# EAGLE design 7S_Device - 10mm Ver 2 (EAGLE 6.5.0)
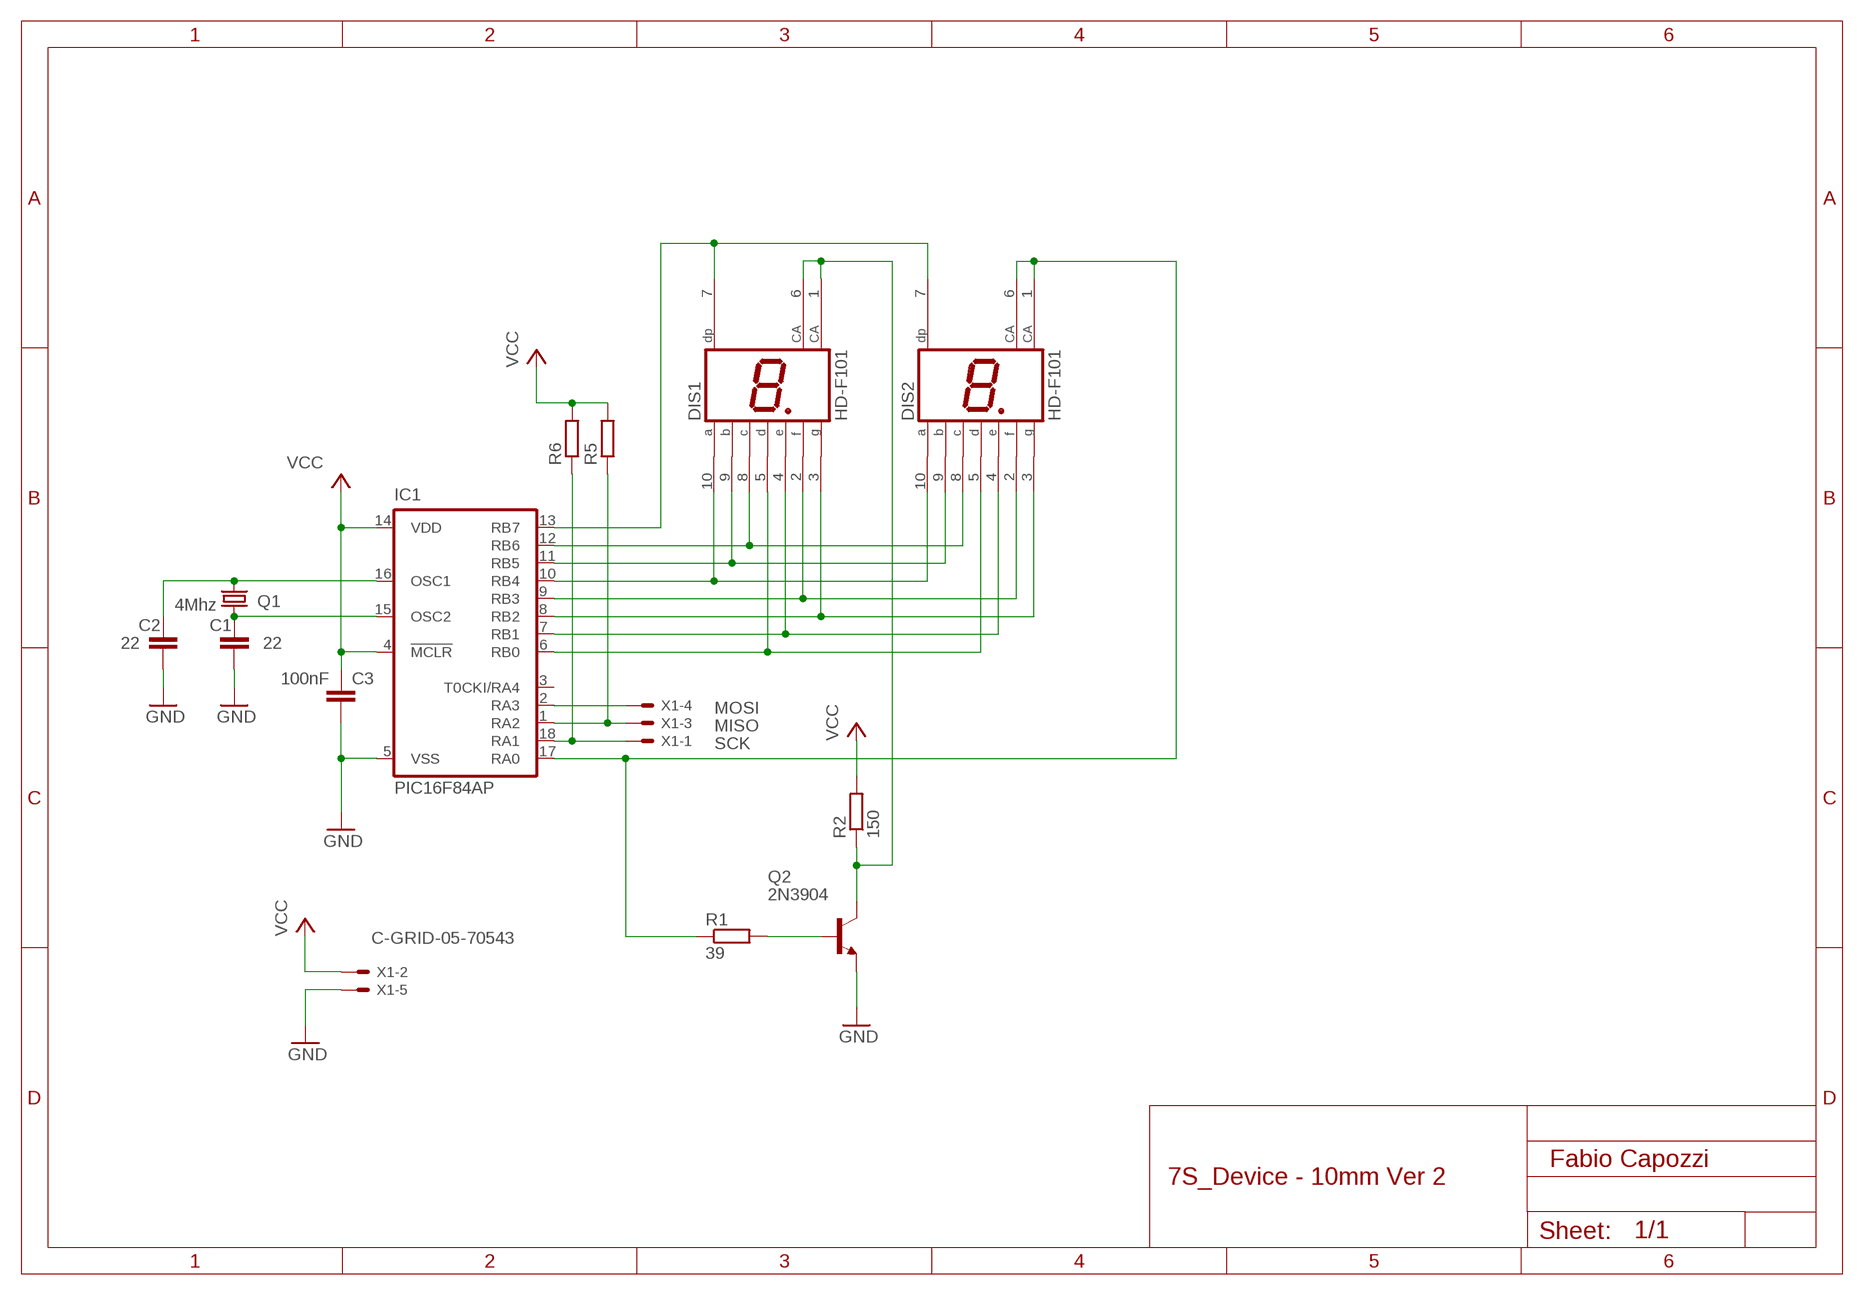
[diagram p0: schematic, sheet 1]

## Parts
C1  22  C5/2.5  [C5B2.5]
C2  22  C5/2.5  [C5B2.5]
C3  100nF  C5/2.5  [C5B2.5]
DIS1  HD-F101  [HDSP-E]
DIS2  HD-F101  [HDSP-E]
IC1  PIC16F84AP  [DIL18]
Q1  4Mhz  CRYSTALHC49U-V  [HC49U-V]
Q2  2N3904  BC489  [TO92-EBC]
R1  39  R-EU_0204/7  [0204/7]
R2  150  R-EU_0204/7  [0204/7]
R5  R-EU_0204/7  [0204/7]
R6  R-EU_0204/7  [0204/7]
X1  C-GRID-05-70543  [70543-05]

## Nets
GND: C1.2 C2.2 C3.2 IC1.5(VSS) Q2.E X1.5
N$1: C2.1 IC1.16(OSC1) Q1.2
N$2: C1.1 IC1.15(OSC2) Q1.1
N$3: DIS1.5(D) DIS2.5(D) IC1.6(RB0)
N$4: DIS1.4(E) DIS2.4(E) IC1.7(RB1)
N$5: DIS1.3(G) DIS2.3(G) IC1.8(RB2)
N$6: DIS1.2(F) DIS2.2(F) IC1.9(RB3)
N$7: DIS1.10(A) DIS2.10(A) IC1.10(RB4)
N$8: DIS1.9(B) DIS2.9(B) IC1.11(RB5)
N$9: DIS1.8(C) DIS2.8(C) IC1.12(RB6)
N$10: DIS1.7(DP) DIS2.7(DP) IC1.13(RB7)
N$11: DIS2.1(CA) DIS2.6(CA) IC1.17(RA0) R1.1
N$12: Q2.B R1.2
N$13: DIS1.1(CA) DIS1.6(CA) Q2.C R2.1
N$15: IC1.18(RA1) R6.1 X1.1
N$18: IC1.1(RA2) R5.1 X1.3
N$19: IC1.2(RA3) X1.4
VCC: C3.1 IC1.4(!MCLR) IC1.14(VDD) R2.2 R5.2 R6.2 X1.2
Unconnected: IC1.3(T0CKI/RA4)

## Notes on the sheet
- MOSI
- MISO
- SCK
- Fabio Capozzi

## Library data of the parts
C1-C3 = capacitor-wima:C: CAPACITOR
DIS1 DIS2 = display-hp:HD-F101: LED DISPLAY 1-character 7 segment, decimal point right; OC_FARNELL: unknown; OC_NEWARK: unknown
IC1 = microchip:PIC16F8*: MICROCONTROLLER 8-Bit PIC16F8X Family - CMOS Flash/EEPROM Pin Compatible : PIC16F83, PIC16CR83, PIC16F84A, PIC16CR84 see also PIC16C*; MF: MICROCHIP; MPN: PIC16F84A-04I/P; OC_FARNELL: 9760865; OC_NEWARK: 69K7635
Q1 = crystal:CRYSTAL: CRYSTAL; OC_FARNELL: 1666969; OC_NEWARK: unknown
Q2 = transistor-npn:BC489*: NPN Transistor
R1 R2 R5 R6 = rcl:R-EU_: RESISTOR, European symbol
X1 = con-molex:C-GRID-05: CONNECTOR wire to board 2.54 mm (0.100") pitch header; OC_FARNELL: unknown; OC_NEWARK: unknown

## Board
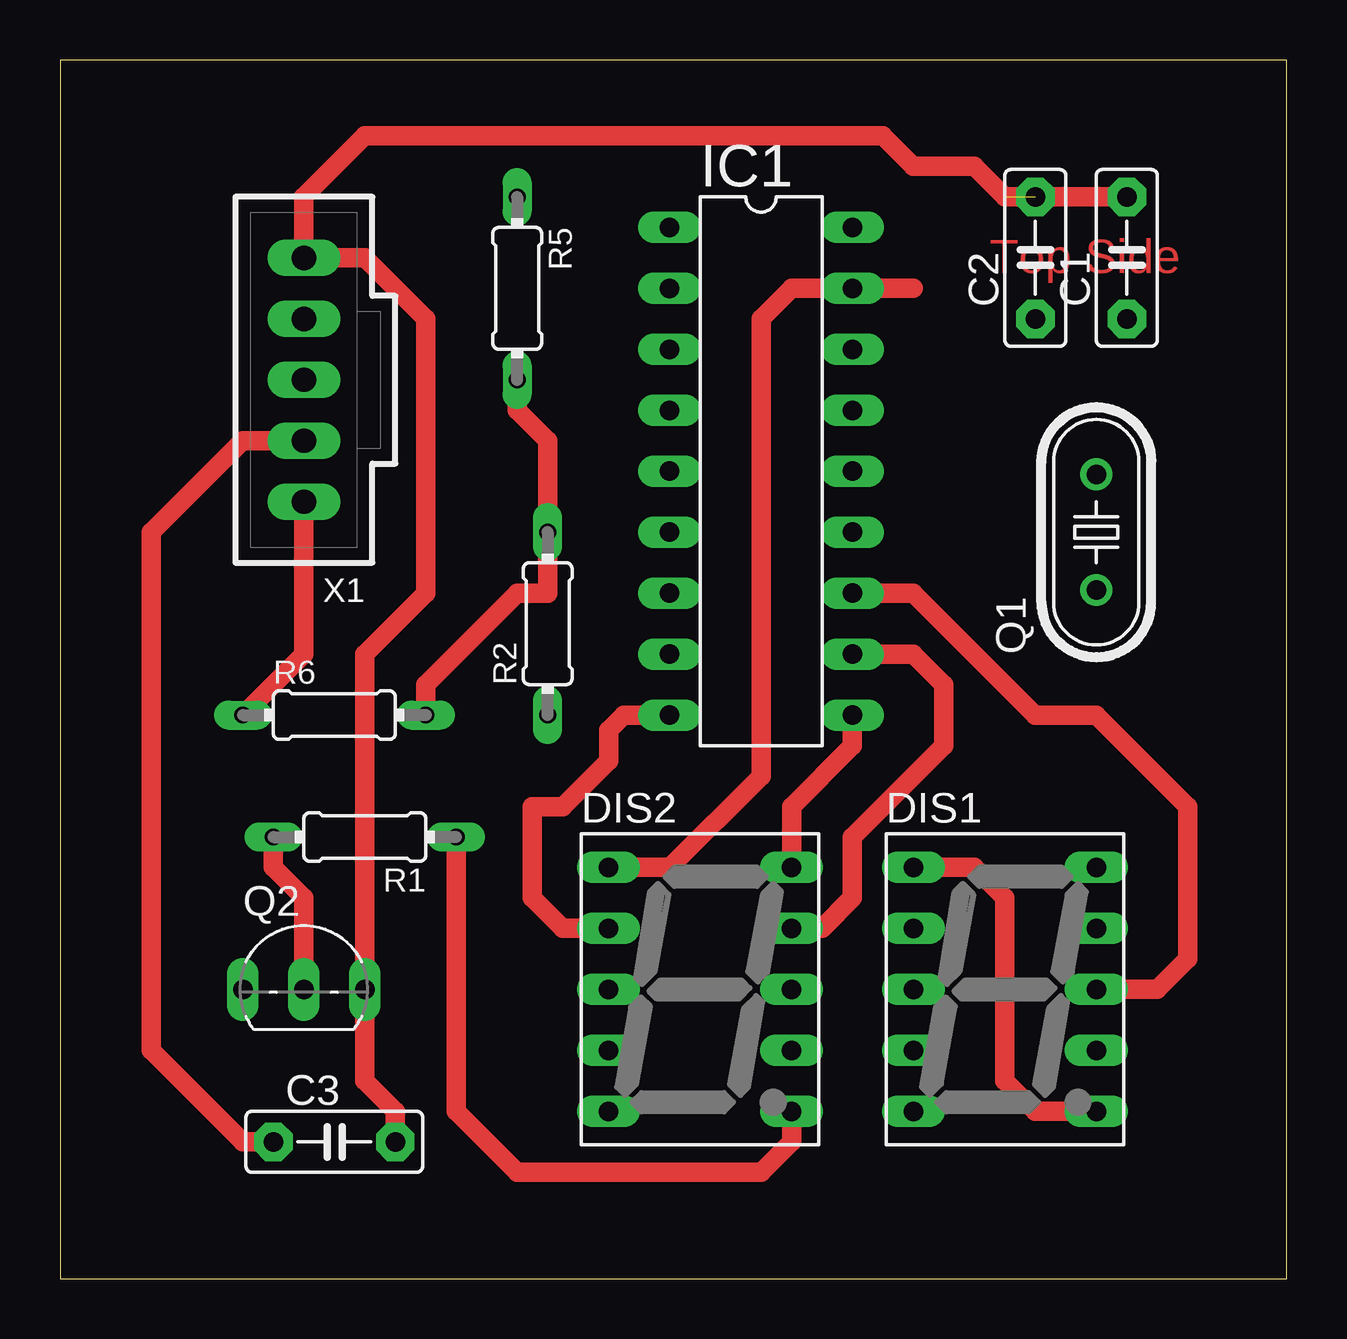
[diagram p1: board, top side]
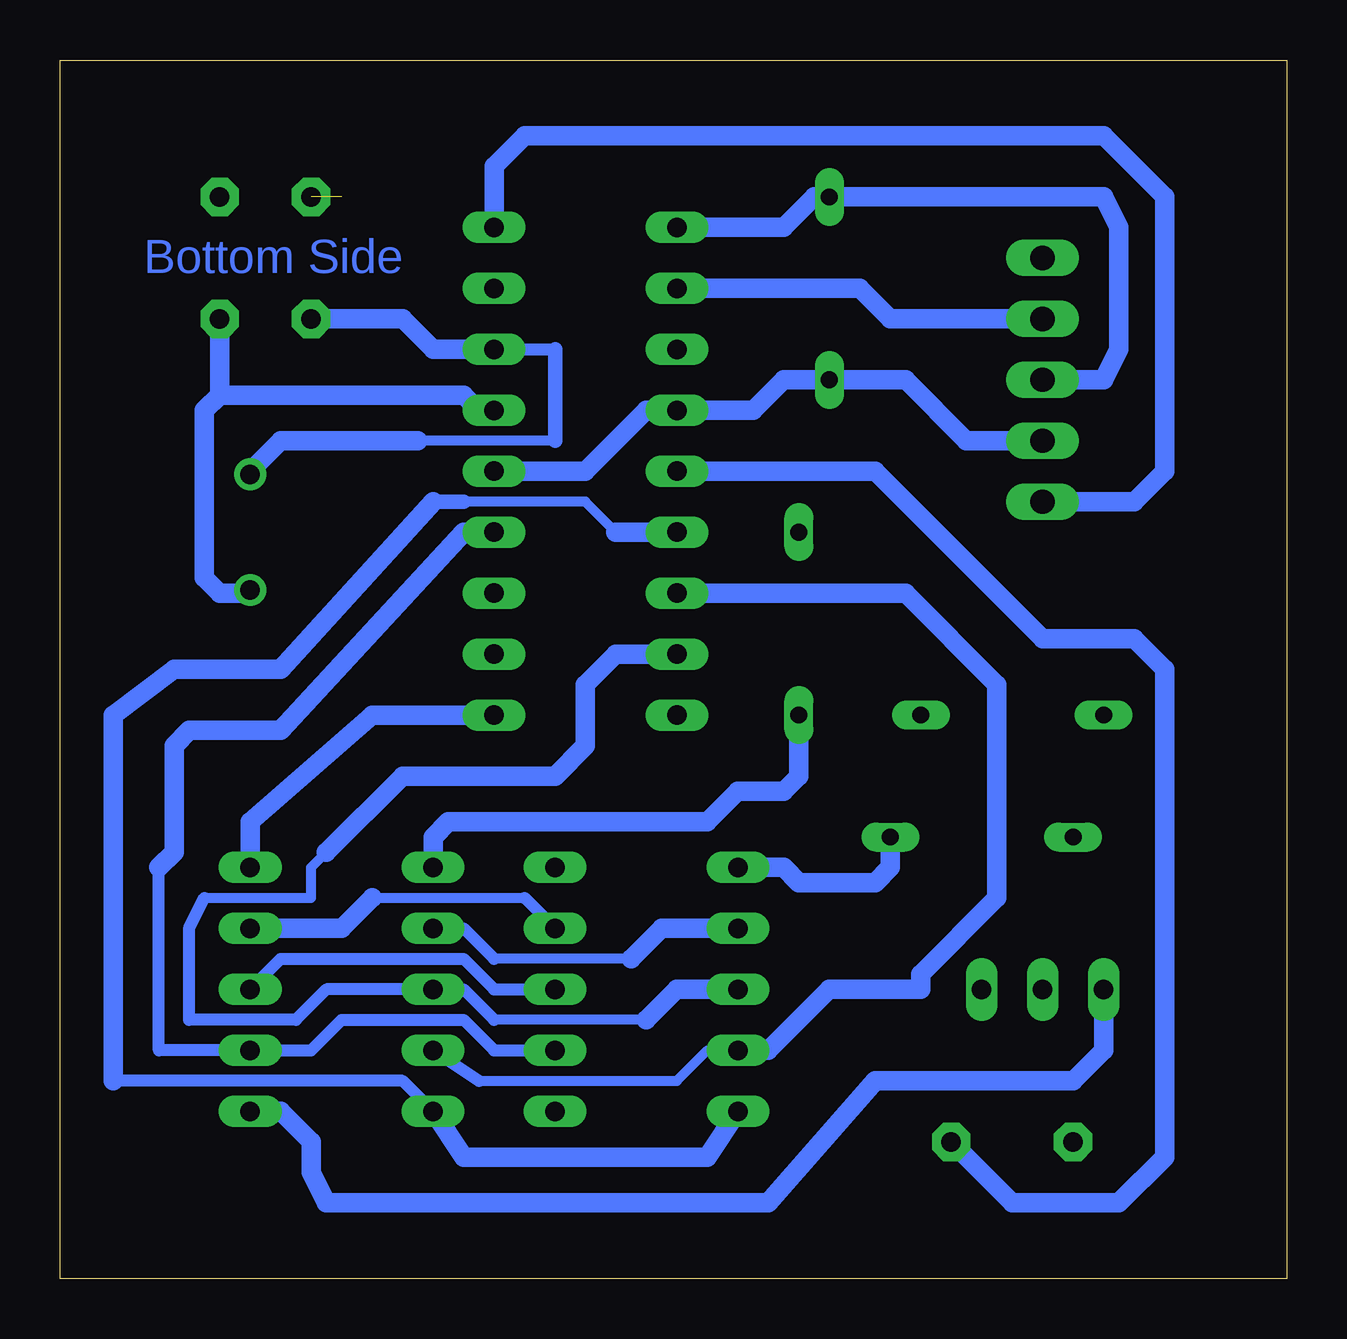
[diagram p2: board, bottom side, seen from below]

Size 51.11 x 50.79 mm. Coordinates in mm from the lower left corner, seen from the top.
Outline: 0,0 51.11,0 51.11,50.79 0,50.79 0,0
Copper layers (1*16): Top 0.035mm / dielectric 1.5mm / Bottom 0.035mm
Design rules "default *": minimum track width 20mil, minimum drill 24mil, track to track 8mil, track to pad 8mil, pad to pad 8mil, via to via 8mil, smd to smd 8mil, copper to edge 40mil, drill to drill 8mil, minimum pad ring 10mil, minimum via ring 8mil, stop-mask expansion 4mil, vias tented up to drill 0mil, thermal gap 10mil
tRestrict: area 40.6,26 to 45.7,36.2; area 26.7,22.2 to 31.8,45.1; area 36.8,5.7 to 41.9,18.4; area 24.1,5.7 to 29.2,18.4

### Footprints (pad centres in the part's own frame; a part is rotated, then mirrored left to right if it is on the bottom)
C5B2.5 = drill 0.813 pad 1.6 octagon: 1 -2.54,0; 2 2.54,0
HDSP-E = drill 0.813 long: 1 -3.81,5.08; 2 -3.81,2.54; 3 -3.81,0; 4 -3.81,-2.54; 5 -3.81,-5.08; 6 3.81,-5.08; 7 3.81,-2.54; 8 3.81,0; 9 3.81,2.54; 10 3.81,5.08
DIL18 = drill 0.813 long: 1 -10.16,-3.81; 2 -7.62,-3.81; 3 -5.08,-3.81; 4 -2.54,-3.81; 5 0,-3.81; 6 2.54,-3.81; 7 5.08,-3.81; 8 7.62,-3.81; 9 10.16,-3.81; 10 10.16,3.81; 11 7.62,3.81; 12 5.08,3.81; 13 2.54,3.81; 14 0,3.81; 15 -2.54,3.81; 16 -5.08,3.81; 17 -7.62,3.81; 18 -10.16,3.81
HC49U-V = drill 0.813: 1 -2.413,0; 2 2.413,0
TO92-EBC = drill 0.813 long: B 0,-1.27; C -2.54,-1.27; E 2.54,-1.27
0204/7 = drill 0.7 pad 1.016 long: 1 -3.81,0; 2 3.81,0
70543-05 = drill 1.016 long: 1 -5.08,0; 2 -2.54,0; 3 0,0; 4 2.54,0; 5 5.08,0

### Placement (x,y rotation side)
C1  44.45,42.54 90 top
C2  40.64,42.54 90 top
C3  11.43,5.71 0 top
DIS1  39.37,12.06 0 top
DIS2  26.67,12.06 0 top
IC1  29.21,33.66 270 top
Q1  43.18,31.12 90 top
Q2  10.16,13.33 0 top
R1  12.7,18.42 180 top
R2  20.32,27.31 90 top
R5  19.05,41.27 270 top
R6  11.43,23.5 0 top
X1  10.16,37.46 90 top

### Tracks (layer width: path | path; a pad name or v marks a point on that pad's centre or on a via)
GND  (1 unrouted)
  Top 0.813: C3.2 13.97,6.98 12.7,8.26 Q2.E 12.7,26.04 15.24,28.58 15.24,40 12.7,42.54 X1.5 10.16,45.09 12.7,47.62 34.29,47.62 35.56,46.35 38.1,46.35 39.37,45.09 C1.2
  Bottom 0.813: C3.2 11.43,3.17 6.98,3.17 5.08,5.08 5.08,25.4 6.35,26.67 10.16,26.67 17.14,33.66 IC1.5
N$1
  Bottom 0.406: 30.48,34.92 36.2,34.92
  Bottom 0.508: IC1.16 30.48,38.73 | 43.18,33.66 Q1.2
  Bottom 0.61: 30.48,38.73 30.48,34.92
  Bottom 0.813: 43.18,33.66 41.91,34.92 36.2,34.92 | IC1.16 35.56,38.73 36.83,40 C2.1
N$2
  Bottom 0.813: IC1.15 33.66,36.2 34.29,36.83 44.45,36.83 | C1.1 44.45,36.83 | 44.45,36.83 45.09,36.2 45.09,29.21 44.45,28.58 43.31,28.58 Q1.1
N$3
  Bottom 0.406: 27.94,31.12 29.21,32.38 34.29,32.38
  Bottom 0.508: 48.9,8.26 36.83,8.26 DIS1.5
  Bottom 0.61: 34.29,32.38 35.56,32.38
  Bottom 0.813: DIS2.5 24.13,5.08 34.29,5.08 DIS1.5 | 35.56,32.38 41.91,25.4 46.36,25.4 48.9,23.5 48.9,8.26 | IC1.6 27.94,31.12
N$4
  Bottom 0.406: 33.66,8.26 25.4,8.26 24.13,9.53 DIS2.4
  Bottom 0.508: DIS1.4 33.66,8.26
  Bottom 0.813: DIS2.4 21.59,9.53 19.05,12.06 15.24,12.06 15.24,12.7 12.06,15.88 12.06,24.77 15.88,28.58 IC1.7
N$5
  Bottom 0.406: 45.09,15.88 40.64,15.88 40.64,17.15 40.01,17.78 | 26.67,10.79 33.02,10.79
  Bottom 0.508: 33.02,10.79 34.29,12.06 DIS1.3 40.01,12.06 41.27,10.79 45.72,10.79 45.72,14.61 45.09,15.88
  Bottom 0.813: 40.01,17.78 36.83,20.96 30.48,20.96 29.21,22.23 29.21,24.77 27.94,26.04 IC1.8 | DIS2.3 25.4,12.06 26.67,10.79
N$6
  Top 0.813: DIS2.2 20.95,14.61 19.69,15.88 19.69,19.69 20.95,19.69 22.86,21.59 22.86,22.86 23.49,23.5 IC1.9
  Bottom 0.406: 27.3,13.33 33.02,13.33
  Bottom 0.508: 33.02,13.33 34.29,14.61 DIS1.2
  Bottom 0.813: DIS2.2 26.03,14.61 27.3,13.33
N$7
  Top 0.813: DIS2.10 30.48,19.69 33.02,22.23 IC1.10
  Bottom 0.813: IC1.10 38.1,23.5 43.18,19.05 DIS1.10
N$8
  Top 0.813: DIS2.9 31.75,14.61 33.02,15.88 33.02,18.42 36.83,22.23 36.83,24.77 35.56,26.04 IC1.11
  Bottom 0.406: 38.1,15.88 31.75,15.88
  Bottom 0.508: 31.75,15.88 DIS2.9 | DIS1.9 41.91,14.61
  Bottom 0.813: 41.91,14.61 39.37,14.61 38.1,15.88
N$9
  Top 0.813: IC1.12 35.56,28.58 40.64,23.5 43.18,23.5 46.99,19.69 46.99,13.33 45.72,12.06 DIS1.8
  Bottom 0.508: DIS2.8 33.02,12.06 34.29,13.33 41.91,13.33 DIS1.8
N$10
  Bottom 0.508: DIS2.7 33.02,9.53 34.29,10.79 39.37,10.79 40.64,9.53 DIS1.7 46.99,9.53 46.99,17.15
  Bottom 0.813: IC1.13 34.29,31.12 41.91,22.86 45.72,22.86 46.36,22.23 46.36,17.78 46.99,17.15
N$11
  Top 0.813: DIS2.1 25.4,17.15 29.21,20.96 29.21,40 30.48,41.27 IC1.17 35.56,41.27 | R1.1 16.51,6.98 19.05,4.45 29.21,4.45 30.48,5.71 DIS2.6
  Bottom 0.813: DIS2.1 20.95,17.15 20.32,16.51 17.14,16.51 16.51,17.15 R1.1
N$12
  Top 0.813: R1.2 8.89,17.15 10.16,15.88 Q2.B
N$13
  Top 0.813: DIS1.1 38.1,17.15 39.37,15.88 39.37,8.26 40.64,6.98 DIS1.6
  Bottom 0.813: Q2.C 7.62,9.53 8.89,8.26 17.14,8.26 21.59,3.17 40.01,3.17 40.64,4.45 40.64,5.71 41.91,6.98 DIS1.6 | R2.1 20.32,20.96 20.95,20.32 22.86,20.32 24.13,19.05 34.92,19.05 35.56,18.42 DIS1.1
N$15
  Top 0.813: X1.1 10.16,26.04 R6.1
  Bottom 0.813: IC1.18 33.02,46.35 31.75,47.62 7.62,47.62 5.08,45.09 5.08,33.66 6.35,32.38 X1.1
N$18
  Bottom 0.813: X1.3 7.62,37.46 6.98,38.73 6.98,43.81 7.62,45.09 R5.1 19.69,45.09 20.95,43.81 IC1.1
N$19
  Bottom 0.813: X1.4 16.51,40 17.78,41.27 IC1.2
VCC
  Top 0.813: X1.2 7.62,34.92 3.81,31.12 3.81,9.53 7.62,5.71 C3.1 | R6.2 15.24,24.77 19.05,28.58 20.32,28.58 R2.2 20.32,34.92 19.05,36.2 R5.2
  Bottom 0.813: IC1.14 29.21,33.66 26.67,36.2 IC1.4 22.23,36.2 20.95,37.46 R5.2 15.88,37.46 13.34,34.92 X1.2

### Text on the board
Top: Top Side
Bottom: Bottom Side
